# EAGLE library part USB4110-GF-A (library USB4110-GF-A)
CONN USB 2.0 TYPE-C R/A SMT Source: Datasheet
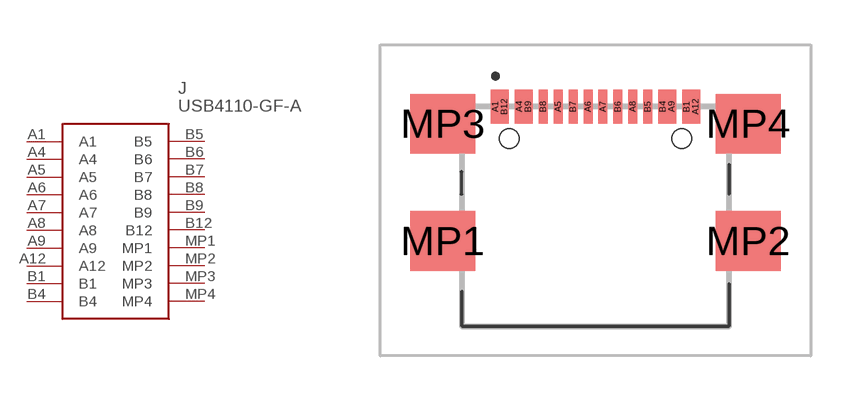
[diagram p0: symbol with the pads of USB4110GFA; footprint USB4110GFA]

Designator prefix J

## USB4110-GF-A (Description: CONN USB 2.0 TYPE-C R/A SMT; Height: 3.26mm; Manufacturer_Name: GCT (GLOBAL CONNECTOR TECHNOLOGY); Manufacturer_Part_Number: USB4110-GF-A; Mouser_Part_Number: 640-USB4110-GF-A; Mouser_Price-Stock: https://www.mouser.co.uk/ProductDetail/GCT/USB4110-GF-A?qs=KUoIvG%2F9IlYiZvIXQjyJeA%3D%3D)  [USB4110GFA]
A1  A1
A4  A4
A5  A5
A6  A6
A7  A7
A8  A8
A9  A9
A12  A12
B1  B1
B4  B4
B5  B5
B6  B6
B7  B7
B8  B8
B9  B9
B12  B12
MP1  MP1
MP2  MP2
MP3  MP3
MP4  MP4

## Footprint USB4110GFA (pad centres in mm)
USB4110-GF-A-1
smd 0.3 x 1.15: A1 -3.35,3.678; A4 -2.55,3.678; A5 -1.25,3.678; A6 -0.25,3.678; A7 0.25,3.678; A8 1.25,3.678; A9 2.55,3.678; A12 3.35,3.678; B1 3.05,3.678; B4 2.25,3.678; B5 1.75,3.678; B6 0.75,3.678; B7 -0.75,3.678; B8 -1.75,3.678; B9 -2.25,3.678; B12 -3.05,3.678
smd 2.18 x 2: MP1 -5.11,-0.827; MP2 5.11,-0.827; MP3 -5.11,3.103; MP4 5.11,3.103
hole 0.65 at -2.89,2.603
hole 0.65 at 2.89,2.603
